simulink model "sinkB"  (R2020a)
settings: Solver=ode45  StartTime=0.0  StopTime=3000  RelTol=1e-3  EnableMultiTasking=on
InitFcn:
  | init_sink
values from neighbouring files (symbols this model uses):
  A = 0.1    [init_sink.m]    (also in init_waermeleit2.m = diag(-2*ones(N+1,1)) + diag(ones(N,1), 1) + diag(ones(N,1), )
  c1 = 1e7    (= 10000000)    [init_sink.m]    (also in init_waermeleit1.m = 0.002908; init_waermeleit2.m = 0.0727)
  c2 = 3e14    (= 300000000000000)    [init_sink.m]
  g = 9.81    [init_sink.m]
  rho = 1000    [init_sink.m]

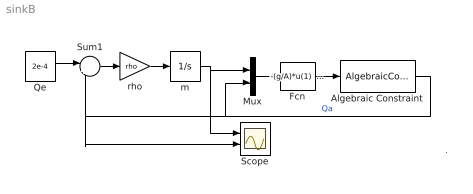
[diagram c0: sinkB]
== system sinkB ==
  note: .
  Algebraic Constraint : AlgebraicConstraint
  Fcn : Fcn  Expr="-(g/A)*u(1)  + c1*u(2) + c2*u(2)^3"
  Mux : Mux  Inputs=2
  Qe : Constant  Value=2e-4
  Scope : Scope  NumInputPorts=2
  Sum1 : Sum  Inputs=|+-  SaturateOnIntegerOverflow=on
  m : Integrator  InitialCondition=10
  rho : Gain  Gain=rho
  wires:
  Qe/1 -> Sum1/1
  Sum1/1 -> rho/1
  m/1 -> Scope/1, Mux/1
  Mux/1 -> Fcn/1
  Fcn/1 -> Algebraic Constraint/1
  Algebraic Constraint/1 -> Scope/2, Sum1/2, Mux/2  "Qa"
  rho/1 -> m/1
